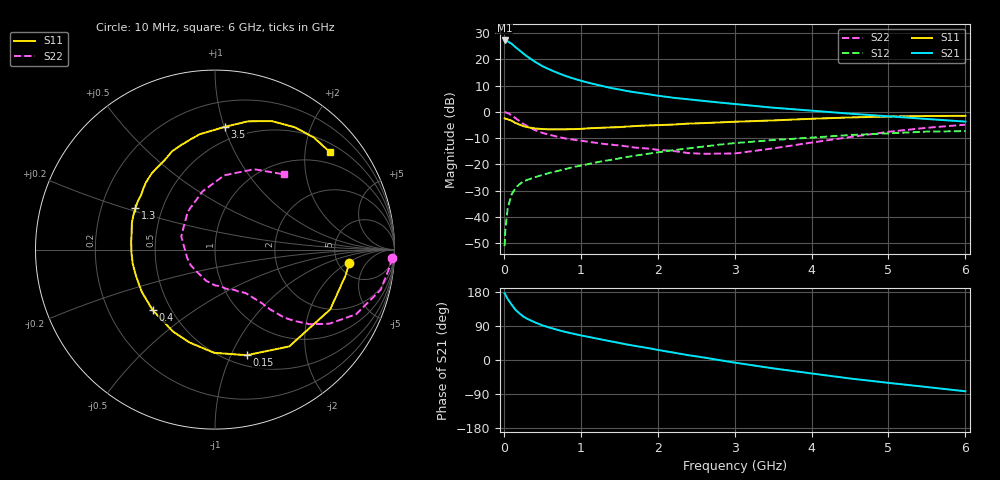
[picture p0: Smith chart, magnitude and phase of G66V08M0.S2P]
! SIEMENS Small Signal Semiconductors
! BFG193
! Si NPN RF Bipolar Junction Transistor in SOT223
! VCE = 6 V  IC = 8 mA
! Common Emitter S-Parameters:  August  1996
# GHz  S  MA  R  50
!  f  S11  S21  S12  S22
! GHz  MAG  ANG  MAG  ANG  MAG  ANG  MAG  ANG
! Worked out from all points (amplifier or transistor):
!   36 points, 10 MHz to 6 GHz, reference 50 ohm
!   highest |S21| = 27.1 dB at 10 MHz (marker M1)
!   |S21| within 3 dB of that: start of sweep to 171.1 MHz
!   unconditionally stable (mu >= 1): 968.7 MHz to 2.473 GHz
!   at 250 MHz: K = 0.46, MSG = 24.4 dB, |S12| = -26.6 dB
!   at 1.4 GHz: K = 1.07, MAG = 12.0 dB, |S12| = -18.2 dB
!   at 6 GHz: K = 0.86, MSG = 1.8 dB, |S12| = -7.3 dB
!   S11 on the Smith chart (normalised r, x): 10 MHz: 6.32, -2.18; 150 MHz: 0.61, -1.15; 400 MHz: 0.40, -0.35; 1.3 GHz: 0.35, +0.22; 3.5 GHz: 0.39, +1.01; 6 GHz: 0.70, +2.57
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0.01  0.7528 -5.7  22.73 175.9  0.0028 93.6  0.9854 -2.7
0.02  0.7413 -11.3  22.68 172.9  0.0059 81.7  0.9791 -5.5
0.05  0.7233 -27.4  21.88 160.9  0.0146 77.9  0.9501 -13.6
0.1  0.6799 -52.5  19.72 146.5  0.0267 66.5  0.8651 -24.6
0.15  0.6144 -73.3  17.04 132.7  0.0356 58.5  0.7597 -32.9
0.2  0.5749 -90.5  14.88 123.5  0.0418 54.2  0.6742 -38.1
0.25  0.5368 -105.3  12.93 115.3  0.047 50.4  0.5955 -41.9
0.3  0.5134 -117.0  11.36 109.1  0.0505 49.4  0.5396 -44.5
0.4  0.4842 -135.8  9.041 99.7  0.0571 47.2  0.4532 -47.3
0.5  0.471 -150.1  7.409 91.5  0.063 46.3  0.3988 -48.8
0.6  0.4641 -161.2  6.321 85.1  0.0696 47.1  0.3637 -50.3
0.7  0.4653 -170.4  5.499 79.4  0.0751 47.7  0.3358 -52.0
0.9  0.4693 174.3  4.323 69.5  0.0892 47.5  0.2958 -54.8
1.1  0.4859 162.5  3.573 61.0  0.1019 47.3  0.2701 -60.4
1.3  0.4999 152.4  3.05 52.9  0.1164 46.0  0.2457 -65.3
1.6  0.5252 139.4  2.49 40.9  0.1388 43.0  0.2203 -76.4
2.2  0.5725 119.2  1.855 19.7  0.1864 34.5  0.1809 -105.6
2.8  0.6296 102.4  1.504 -0.2  0.2377 23.7  0.1608 -147.1
3.5  0.6867 85.3  1.199 -22.0  0.291 8.2  0.202 158.5
4.5  0.7826 66.2  0.923 -48.8  0.363 -11.7  0.3316 102.1
5.5  0.8327 48.6  0.732 -71.4  0.4216 -36.6  0.4981 64.0
6  0.8396 40.2  0.652 -82.5  0.4301 -50.9  0.5698 47.3
